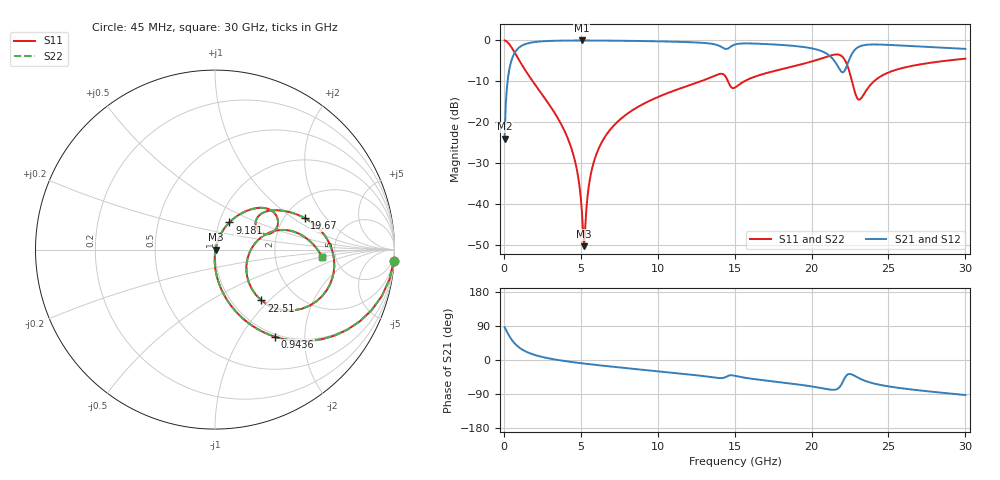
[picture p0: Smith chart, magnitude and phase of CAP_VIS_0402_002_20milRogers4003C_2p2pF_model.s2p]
! S-parameter model data by Modelithics Inc.  support@modelithics.com  813-866-6335  Tampa FL USA
! S-Parameter data specifications:
! Substrate: 20-mil Rogers 4003C, substrate thickness, H=0.508mm, Dielectric constant, Er=3.75
! PCB Mounting Pad Footprint: Pad width, PadW=0.50mm , Pad length, PadL=0.50mm , Pad gap, PadG (edge-to-edge)=0.40mm , Reference planes=1.4mm apart
! Created Wed Nov 18 12:44:38 2015
# hz S ma R 50
! 2 Port Network Data from SP1.SP block
! freq  magS11  angS11  magS21  angS21  magS12  angS12  magS22  angS22
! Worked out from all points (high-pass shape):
!   401 points, 45 MHz to 30 GHz, reference 50 ohm
!   highest |S21| = -0.03 dB at 5.062 GHz (marker M1); lowest = -24.0 dB at 45 MHz (marker M2)
!   |S21| within 3 dB of the highest: 702.4 MHz to 20.88 GHz (20.18 GHz wide, 187 % of centre); 22.67 GHz to end of sweep
!   lowest |S11| = -50.3 dB at 5.212 GHz (marker M3), VSWR 1.01, Z = 50.3 - j0.0242 ohm
!   |S11| at or under -10 dB: 1.871 GHz to 12.79 GHz (10.92 GHz wide, 149 % of centre); 14.56 GHz to 15.63 GHz (1.069 GHz wide, 7.08 % of centre); 22.63 GHz to 24.06 GHz (1.432 GHz wide, 6.13 % of centre)
!   |S22| runs from -50.3 to 0.0 dB; largest |S21 - S12| = 0
!   S11 on the Smith chart (normalised r, x): 45 MHz: 1, -31; 943.6 MHz: 0.96, -1.44; 9.181 GHz: 1.12, +0.35; 19.67 GHz: 2.56, +1.25; 22.51 GHz: 1.35, -0.90; 30 GHz: 3.91, -0.47
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4.5e7  0.998 -3.7  0.06276 86.3  0.06276 86.3  0.998 -3.7
4.194375e8  0.8611 -31.3  0.5079 58.7  0.5079 58.7  0.8611 -31.3
9.4365e8  0.5912 -55.4  0.8054 34.5  0.8054 34.5  0.5912 -55.4
1.992075e9  0.2934 -76.2  0.9541 13.5  0.9541 13.5  0.2934 -76.2
4.088925e9  0.06758 -91.3  0.9949 -3.5  0.9949 -3.5  0.06758 -91.3
4.688025e9  0.0294 -91.2  0.9966 -6.8  0.9966 -6.8  0.0294 -91.2
5.062462e9  0.008416 -77.9  0.9968 -8.7  0.9968 -8.7  0.008416 -77.9
5.212238e9  0.003039 -4.5  0.9968 -9.4  0.9968 -9.4  0.003039 -4.5
5.661562e9  0.02364 70.7  0.9964 -11.6  0.9964 -11.6  0.02364 70.7
6.260662e9  0.05214 72.0  0.9951 -14.3  0.9951 -14.3  0.05214 72.0
9.181275e9  0.1715 62.1  0.9805 -26.4  0.9805 -26.4  0.1715 62.1
1.007992e10  0.2054 58.6  0.9735 -30.0  0.9735 -30.0  0.2054 58.6
1.404896e10  0.3891 31.1  0.8491 -47.8  0.8491 -47.8  0.3891 31.1
1.50225e10  0.2648 31.4  0.8902 -41.8  0.8902 -41.8  0.2648 31.4
1.966552e10  0.5296 19.4  0.8203 -67.6  0.8203 -67.6  0.5296 19.4
2.003996e10  0.5541 16.4  0.7969 -70.0  0.7969 -70.0  0.5541 16.4
2.16126e10  0.6732 -11.0  0.5173 -77.5  0.5173 -77.5  0.6732 -11.0
2.206192e10  0.6137 -30.5  0.4075 -54.8  0.4075 -54.8  0.6137 -30.5
2.251125e10  0.383 -47.6  0.6204 -37.0  0.6204 -37.0  0.383 -47.6
2.311035e10  0.1882 -12.4  0.841 -48.5  0.841 -48.5  0.1882 -12.4
2.505742e10  0.4088 15.5  0.8797 -70.0  0.8797 -70.0  0.4088 15.5
3e10  0.5976 -3.7  0.7871 -92.4  0.7871 -92.4  0.5976 -3.7
